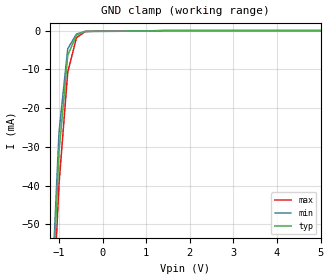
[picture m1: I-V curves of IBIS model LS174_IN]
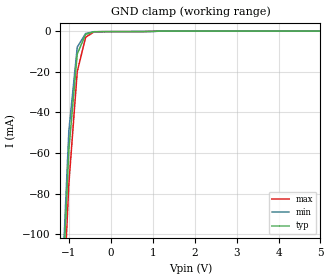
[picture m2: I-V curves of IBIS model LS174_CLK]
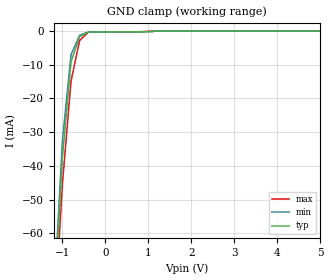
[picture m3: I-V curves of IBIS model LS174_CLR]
|   TEXAS INSTRUMENTS INCORPORATED
|   Standard Linear and Logic Group
|   IBIS Model of SN74LS174
|   HEX/QUADRUPLE D-TYPE FLIP-FLOPS WITH CLEAR
|   SOIC 16-pin (D), PDIP 16-pin (N)
[IBIS Ver]   3.2
[Comment Char]  |_char
[File Name]   sn74ls174.ibs
[File Rev]   1.2 | c_die
[Date]   Nov. 17, 2004
[Source]   File originated at Texas Instruments, Inc.
[Notes]   The following is a sample IBIS file for the SN74LS174.
   - FILE REV HISTORY
   - 3.1 Re-Release IBIS file on 11/19/04
   - Power clamp data deleted as there is no power-clamp diode
   - All test data contained in this file are derived from
   actual measurements.
   - The measurement used NS package.
   - File created by Nobuhisa Ohtsubo, SLL Product Engineering.
[Disclaimer] Property of Texas Instruments Incorporated. Unauthorized
   reproduction and/or distribution is strictly prohibited.
   This product is protected under copyright law.
   Created 2000, (C) Copyright 2000, Texas Instruments Inc.,
   All Rights Reserved.
   UNLESS THERE IS A SIGNED, WRITTEN AGREEMENT TO THE
   CONTRARY, TEXAS INSTRUMENTS () IS PROVIDING THE IBIS
   MODELS AND WITHOUT ANY WARRANTY, EXPRESSED OR
   IMPLIED. TI assumes no liability for:
   1) the accuracy of the IBIS models provided to your
   company;
   2) the proper functioning of these IBIS Models in your
   design or for any resulting applications; or
   3) infringement of patents, copyrights or intellectual
   property rights resulting from your use of these IBIS
   models.
   TI provides IBIS Models as a service to our customers.
   You and your company shall not distribute, sell or give
   these models to anyone else without prior written
   permission from TI.
   TI reserves the right to make changes to our products or
   to discontinue any semiconductor product or service
   without notice, and advises our customers to obtain the
   latest version of relevant information to verify, before
   placing orders, that the information being relied on is
   current.
   Please be aware that your receipt and use of the IBIS
   information provided shall serve as acceptance of these
   terms and conditions. If you do not accept these terms,
   you should return or destroy the IBIS models and any
   other accompanying information immediately.
| Component LS174_D
[Component]   LS174_D
[Manufacturer]  Texas Instruments, Inc.
[Package]
|   typ   min   max
R_pkg   0.039   0.028   0.049
L_pkg   3.453nH   2.350nH   4.375nH
C_pkg   0.521pF   0.254pF   0.708pF
[Pin]   signal_name   model_name   R_pin   L_pin   C_pin
1   NCLR   LS174_CLR   0.042   4.336nH   0.703pF
2   1Q   LS174_OUT   0.049   3.778nH   0.634pF
3   1D   LS174_IN   0.028   3.449nH   0.518pF
4   2D   LS174_IN   0.029   2.393nH   0.254pF
5   2Q   LS174_OUT   0.028   2.350nH   0.264pF
6   3D   LS174_IN   0.048   3.312nH   0.483pF
7   3Q   LS174_OUT   0.043   3.629nH   0.604pF
8   GND   GND   0.044   4.375nH   0.708pF
9   CLK   LS174_CLK   0.042   4.336nH   0.703pF
10   4Q   LS174_OUT   0.049   3.778nH   0.634pF
11   4D   LS174_IN   0.028   3.449nH   0.518pF
12   5Q   LS174_OUT   0.029   2.393nH   0.255pF
13   5D   LS174_IN   0.028   2.350nH   0.264pF
14   6D   LS174_IN   0.048   3.312nH   0.483pF
15   6Q   LS174_OUT   0.043   3.629nH   0.604pF
16   VCC   POWER   0.044   4.375nH   0.708pF
| Component LS174_N
[Component]   LS174_N
[Manufacturer]  Texas Instruments, Inc.
[Package]
|   typ   min   max
R_pkg   5.600e-02   5.200e-02   6.300e-02
L_pkg   7.637e-09   5.451e-09   1.053e-08
C_pkg   5.280e-13   3.350e-13   8.930e-13
[Pin]   signal_name   model_name   R_pin   L_pin   C_pin
1   NCLR   LS174_CLR   5.800e-02   1.053e-08   8.920e-13
2   1Q   LS174_OUT   6.200e-02   8.759e-09   5.350e-13
3   1D   LS174_IN   5.200e-02   7.146e-09   3.870e-13
4   2D   LS174_IN   5.300e-02   5.451e-09   4.080e-13
5   2Q   LS174_OUT   5.300e-02   5.513e-09   3.700e-13
6   3D   LS174_IN   5.300e-02   6.304e-09   3.360e-13
7   3Q   LS174_OUT   5.700e-02   7.830e-09   5.030e-13
8   GND   GND   5.600e-02   9.581e-09   8.050e-13
9   CLK   LS174_CLK   5.800e-02   9.603e-09   8.070e-13
10   4Q   LS174_OUT   6.200e-02   7.864e-09   5.030e-13
11   4D   LS174_IN   5.200e-02   6.295e-09   3.350e-13
12   5Q   LS174_OUT   5.300e-02   5.499e-09   3.560e-13
13   5D   LS174_IN   5.300e-02   5.452e-09   4.040e-13
14   6D   LS174_IN   5.300e-02   7.156e-09   3.870e-13
15   6Q   LS174_OUT   6.300e-02   8.740e-09   5.340e-13
16   VCC   POWER   5.600e-02   1.048e-08   8.930e-13
| Models and submodels in the file (4): LS174_IN (Input), LS174_CLK (Input), LS174_CLR (Input), LS174_OUT (Output)
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|   Model LS174_IN
[Model]   LS174_IN
Model_type  Input
Polarity   Non-Inverting
Vinl = 0.8
Vinh = 2.0
| variable   typ   min   max
C_comp   1.35pf   1.01pf   1.69pf
[Temperature Range]   25   0   70
[Voltage Range]   5.00   4.75   5.25
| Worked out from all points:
|   GND clamp passes 1 mA (typ) near -0.57 V on its own axis
[GND Clamp]
|   Voltage   I(typ)   I(min)   I(max)
-5V       -1.397A    -1.458A    -1.272A
-1.2V     -80.57mA   -75.85mA   -86.65mA
-1V       -31.27mA   -26.24mA   -39.67mA
-800mV    -6.417mA   -4.717mA   -10.78mA
-600mV    -1.146mA   -885.5uA   -1.844mA
-400mV    -212.7uA   -211.4uA   -265.9uA
-200mV    -196.1uA   -201uA     -175.5uA
5V        5.466nA    47.68nA    8.204nA
|   Model LS174_CLK
[Model]   LS174_CLK
Model_type  Input
Polarity   Non-Inverting
Vinl = 0.8
Vinh = 2.0
| variable   typ   min   max
C_comp   1.35pf   1.01pf   1.69pf
[Temperature Range]   25   0   70
[Voltage Range]   5.00   4.75   5.25
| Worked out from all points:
|   GND clamp passes 1 mA (typ) near -0.51 V on its own axis
[GND Clamp]
|   Voltage   I(typ)   I(min)   I(max)
-5V       -2.421A    -2.66A     -2.342A
-1.2V     -151.4mA   -142mA     -164.3mA
-1V       -58.59mA   -49.21mA   -75.26mA
-800mV    -11.29mA   -7.915mA   -20mA
-600mV    -1.611mA   -1.189mA   -3.064mA
-400mV    -311.7uA   -310uA     -383.9uA
-200mV    -290uA     -295.5uA   -265.1uA
5V        4.581nA    4.627nA    16.27nA
|   Model LS174_CLR
[Model]   LS174_CLR
Model_type  Input
Polarity   Inverting
Vinl = 0.8
Vinh = 2.0
| variable   typ   min   max
C_comp   1.35pf   1.01pf   1.69pf
[Temperature Range]   25   0   70
[Voltage Range]   5.00   4.75   5.25
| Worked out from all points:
|   GND clamp passes 1 mA (typ) near -0.51 V on its own axis
[GND Clamp]
|   Voltage   I(typ)   I(min)   I(max)
-5V       -1.16A     -1.307A    -1.092A
-1.2V     -83.5mA    -79.88mA   -88.28mA
-1V       -37.42mA   -32.45mA   -45.42mA
-800mV    -9.07mA    -6.954mA   -14.87mA
-600mV    -1.623mA   -1.236mA   -2.78mA
-400mV    -284.7uA   -284.2uA   -364.8uA
-200mV    -261.7uA   -270.3uA   -234.4uA
1.2V      -2.24uA    -8.78uA    -183.2nA
5V        4.488nA    71.44nA    15.79nA
